(* Logix 5000 Rung export; software revision 16.03 *)

MODULES
   MNETCR : vendor None type None code None
   RemoteENBT_Slot6 : vendor None type None code None
END_MODULES

TYPE MNETCRCONTROL :   // Values used by program for data transfer operation between the module and the processor.
STRUCT
   BootTimer : TIMER;   // Timer used to clear both cold and warm boot requests
   WarmBoot : BOOL;   // Partial reset of the Module.
   ColdBoot : BOOL;   // Full reset of the Module.
   ResetStatus : BOOL;   // Resets module status
   EventCmdTrigger : BOOL;   // Initiates Event Command.
   EventCmdPending : BOOL;   // Allows Event Command.
   ClientID : INT;   // Client ID to poll a server with the Event Command.
   EventCmd : MNETCREVENTCMD;   // Holds Event Command configuration
   CmdControl : MNETCRCMDCONTROL;   // Holds Command Control status
   CmdControlTrigger : BOOL;   // Initiates Command Control.
   CmdControlPending : BOOL;   // Allows CmdControlTriger.
   IPAddress : MNETCRIPADDRESS;   // IP address statistics including triggers
   WriteCmdBits : INT[30];   // Selects individual clients to to activate its commands.
END_STRUCT
END_TYPE

TYPE MNETCRDATA :   // Contains Read Data (data read from the module to the processor) and Write Data (data written from the processor to the module)
STRUCT
   ReadData : INT[600];   // Data read from module
   WriteData : INT[600];   // Data to write to module
END_STRUCT
END_TYPE

TYPE MNETCREVENTCMD :   // Data structure to use for Event message generation.
STRUCT
   IP0 : INT;   // First digit of IP address
   IP1 : INT;   // Second digit of IP address
   IP2 : INT;   // Third digit of IP address
   IP3 : INT;   // Last digit of IP address
   ServPort : INT;   // TCP Service Port number (0-65535), 502 for MBAP, 2000 for MNET
   SlvAddrNode : INT;   // Modbus slave node address (0 to 247)
   DBAddress : INT;   // Module internal database to use with message
   Count : INT;   // Register or data point count
   Swap : INT;   // Swap code to use with functions 3 and 4
   MBFunction : INT;   // Modbus function code for message
   Address : INT;   // Address to interface with in device
END_STRUCT
END_TYPE

TYPE MNETCRIPADDRESS :   // This object holds IP address status with set IP & get IP triggers.
STRUCT
   IPgetTrigger : BOOL;   // Triggers get IP address.
   IPreceived : INT[4];   // Displays received IP address.
   IPsetTrigger : BOOL;   // Triggers set IP address
   IPrequested : INT[4];   // Displays requested IP address
END_STRUCT
END_TYPE

TYPE MNETCRMODULEDEF :   // This defines the whole module which includes all tags used in the program
STRUCT
   DATA : MNETCRDATA;   // Data read from module
   CONTROL : MNETCRCONTROL;   // MNETCR Module control
   STATUS : MNETCRSTATUS;   // Client ,Server Status and blocks status
   UTIL : MNETCRUTIL;   // Block statistics
END_STRUCT
END_TYPE

TYPE MNETCRUTIL :   // Values used by program for data transfer operation between the module and the processor.
STRUCT
   LastRead : INT;   // Index of last read block
   LastWrite : INT;   // Index of last write block
   BlockIndex : INT;   // Computed block offset for data table
   ReadDataSizeGet : INT;   // Gets ReadData Array Length.
   WriteDataSizeGet : INT;   // Gets WriteData Array Length.
   ReadDataBlkCount : INT;   // Holds the value of the Block Counts of the Read Data Array.
   WriteDataBlkCount : INT;   // Holds the value of the Block Counts of the Write Data Array.
   RBTSremainder : INT;   // Holds remainder calculation value from the read array.
   WBTSremainder : INT;   // Holds remainder calculation value from the write array.
   IPgetPending : BOOL;   // Allows setting IP
   IPsetPending : BOOL;   // Allowes getting IP
   InitOutBlkIDLim : INT;   // Block Index Limit for ReadData size of the array
END_STRUCT
END_TYPE

TYPE MNETCRBLOCKSTATS :   // This object is used to store the block transfer statistics for the MVI56-MNETCR module.
STRUCT
   Read : INT;   // Total number of read block transfers
   Write : INT;   // Total number of write block transfers
   Parse : INT;   // Total number of blocks parsed
   Event : INT;   // Total number of event blocks received
   Cmd : INT;   // Total number of command blocks received
   Err : INT;   // Total number of block transfer errors
END_STRUCT
END_TYPE

TYPE MNETCRCLIENTSTATS :   // This object is used to store the port statistics for an MVI56-MNETCR port.
STRUCT
   CmdReq : INT;   // Total number of command list requests sent
   CmdResp : INT;   // Total number of command list responses received
   CmdErr : INT;   // Total number of command list errors
   Requests : INT;   // Total number of requests for port
   Responses : INT;   // Total number of responses for port
   ErrSent : INT;   // Total number of errors sent
   ErrRec : INT;   // Total number of errors received
   CfgErrWord : INT;   // Configuration Error Word
   CurErr : INT;   // Current Error code
   LastErr : INT;   // Last recorded error code
END_STRUCT
END_TYPE

TYPE MNETCRCMDCONTROL :   // MVI56E-MNETCR Command Control
STRUCT
   ClientIDreq : INT;   // Requested Client ID.
   CmdQty : INT;   // Command Quantaty for the Client.
   CmdIndex : INT[16];   // Command Index per client. (0 to 15)
END_STRUCT
END_TYPE

TYPE MNETCRSTATUS :   // This status data is returned on each read block and can be used to detect proper module operation.
STRUCT
   PassCnt : INT;   // Program cycle counter
   BlockStats : MNETCRBLOCKSTATS;   // Block Statistics
   CmdBits : INT[30];   // Client Command Status.
   ClientStatsTrigger : BOOL;   // Get Client Status
   ClientIDReq : INT;   // Client ID requested.
   ClientStatus : MNETCRCLIENTSTATS[30];   // Client Status requests
   ClientIDRec : INT;   // Client ID received.
   CmdErrorList : INT[16];   // Cmd Error List
   ClientStatsPending : BOOL;   // Allows Get Client Status
END_STRUCT
END_TYPE

ADD_ON_INSTRUCTION AOI56MNETCR   (* revision 1.6, vendor ProSoft Technology Inc. *)
// Add-On for MVI56-MNETCR and  MVI56E-MNETCR Modules
// Revision note:
// v1.6 - Fixed copy length from 10 to 1 with client status logic
VAR_IN_OUT
   Connection_Input : INT[42]; {required}   // Input parameters.
   Connection_Output : INT[42]; {required}   // Output parameters.
   MNETCR : MNETCRMODULEDEF; {required}
END_VAR
VAR
   MJFAULTS : DINT[12];
END_VAR

ROUTINE Logic   (* ladder *)
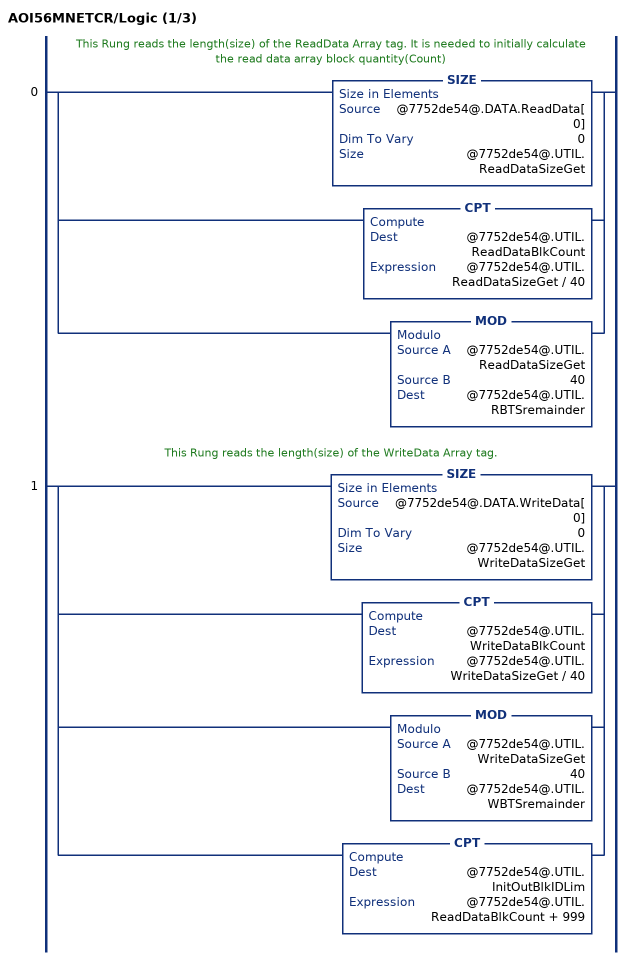
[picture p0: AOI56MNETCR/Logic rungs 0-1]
   // This Rung reads the length(size) of the ReadData Array tag. It is needed to initially calculate the read data array block quantity(Count)
   0: [SIZE(@7752de54@.DATA.ReadData[0],0,@7752de54@.UTIL.ReadDataSizeGet) ,CPT(@7752de54@.UTIL.ReadDataBlkCount,@7752de54@.UTIL.ReadDataSizeGet / 40) ,MOD(@7752de54@.UTIL.ReadDataSizeGet,40,@7752de54@.UTIL.RBTSremainder) ];
   // This Rung reads the length(size) of the WriteData Array tag.
   1: [SIZE(@7752de54@.DATA.WriteData[0],0,@7752de54@.UTIL.WriteDataSizeGet) ,CPT(@7752de54@.UTIL.WriteDataBlkCount,@7752de54@.UTIL.WriteDataSizeGet / 40) ,MOD(@7752de54@.UTIL.WriteDataSizeGet,40,@7752de54@.UTIL.WBTSremainder) ,CPT(@7752de54@.UTIL.InitOutBlkIDLim,@7752de54@.UTIL.ReadDataBlkCount + 999) ];
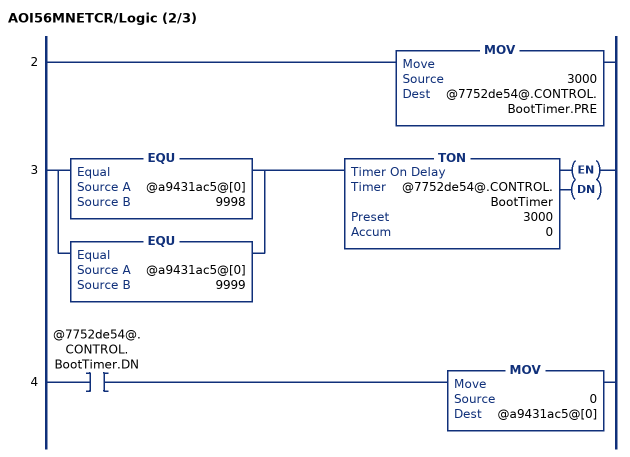
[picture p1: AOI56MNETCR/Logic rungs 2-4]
   2: MOV(3000,@7752de54@.CONTROL.BootTimer.PRE);
   3: [EQU(@a9431ac5@[0],9998) ,EQU(@a9431ac5@[0],9999) ]TON(@7752de54@.CONTROL.BootTimer,3000,0);
   4: XIC(@7752de54@.CONTROL.BootTimer.DN)MOV(0,@a9431ac5@[0]);
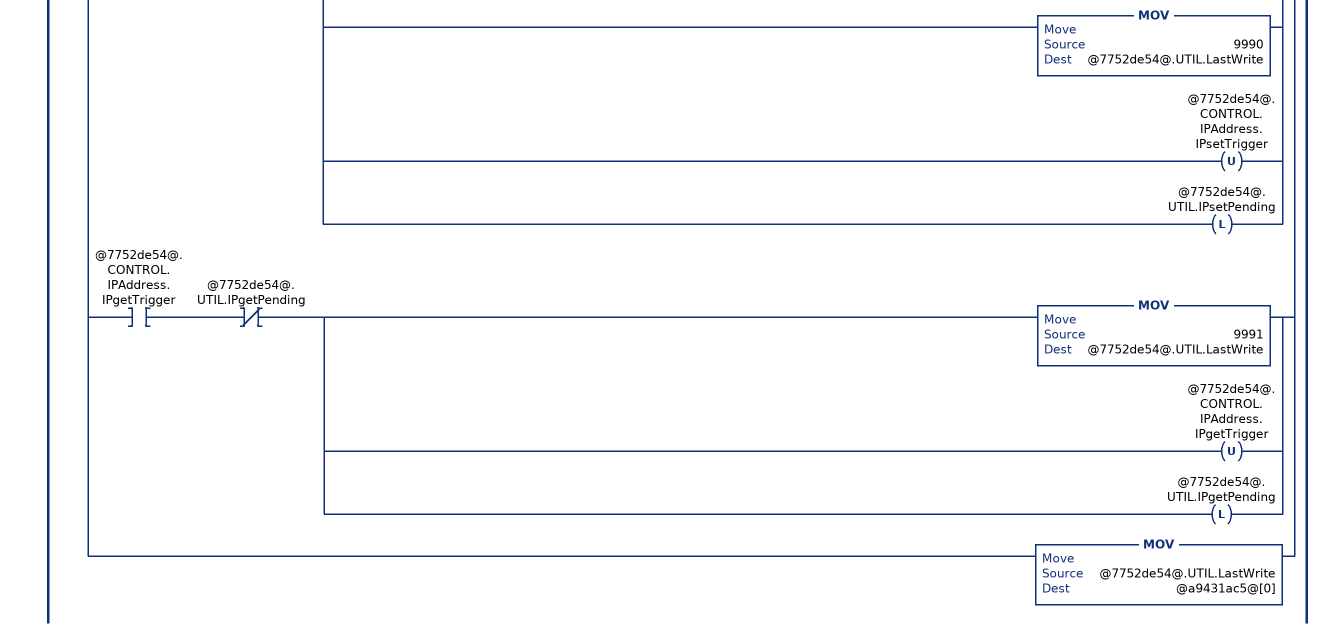
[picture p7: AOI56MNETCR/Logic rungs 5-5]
   // This rung is used to check for a new read block from the MVI56-MNETCR module in slot 1.  If new data is available, the LastRead and Data[41] will not be equal.  This will force the program to call the ReadData subroutine to process the new data received.  After the new data is placed in the Modbus Data Table, the program will send new data to the module using the WriteData subroutine.
   5: NEQ(@0dfc57aa@[41],@7752de54@.UTIL.LastRead)[MOV(@0dfc57aa@[41],@7752de54@.UTIL.LastRead) ,[EQU(-1,@7752de54@.UTIL.LastRead) ,EQU(0,@7752de54@.UTIL.LastRead) ] [MOV(@0dfc57aa@[1],@7752de54@.STATUS.PassCnt) ,COP(@0dfc57aa@[2],@7752de54@.STATUS.BlockStats.Read,6) ,COP(@0dfc57aa@[8],@7752de54@.STATUS.CmdBits[0],30) ] ,GEQ(@7752de54@.UTIL.LastRead,1) [LEQ(@7752de54@.UTIL.LastRead,@7752de54@.UTIL.ReadDataBlkCount) [CPT(@7752de54@.UTIL.BlockIndex,(@7752de54@.UTIL.LastRead - 1) * 40) ,COP(@0dfc57aa@[1],@7752de54@.DATA.ReadData[@7752de54@.UTIL.BlockIndex],40) ] ,CMP(@7752de54@.UTIL.LastRead - @7752de54@.UTIL.ReadDataBlkCount = 1) GRT(@7752de54@.UTIL.RBTSremainder,0) [CPT(@7752de54@.UTIL.BlockIndex,(@7752de54@.UTIL.LastRead - 1) * 40) ,COP(@0dfc57aa@[1],@7752de54@.DATA.ReadData[@7752de54@.UTIL.BlockIndex],@7752de54@.UTIL.RBTSremainder) ] ] ,LIM(2000,@7752de54@.UTIL.LastRead,2029) EQU(@0dfc57aa@[1],1) OTU(@7752de54@.CONTROL.EventCmdPending) ,LIM(3000,@7752de54@.UTIL.LastRead,3029) [MOV(@0dfc57aa@[1],@7752de54@.STATUS.ClientIDRec) ,SUB(@7752de54@.STATUS.ClientIDRec,3000,@7752de54@.STATUS.ClientIDRec) ,COP(@0dfc57aa@[2],@7752de54@.STATUS.ClientStatus[@7752de54@.STATUS.ClientIDRec],1) ,COP(@0dfc57aa@[12],@7752de54@.STATUS.CmdErrorList[0],16) ,OTU(@7752de54@.STATUS.ClientStatsPending) ] ,LIM(5001,@7752de54@.UTIL.LastRead,5016) LIM(1,@0dfc57aa@[1],16) OTU(@7752de54@.CONTROL.CmdControlPending) ,EQU(@7752de54@.UTIL.LastRead,9990) [COP(@0dfc57aa@[1],@7752de54@.CONTROL.IPAddress.IPrequested[0],4) ,OTU(@7752de54@.UTIL.IPsetPending) ] ,EQU(@7752de54@.UTIL.LastRead,9991) [COP(@0dfc57aa@[1],@7752de54@.CONTROL.IPAddress.IPreceived[0],4) ,OTU(@7752de54@.UTIL.IPgetPending) ] ,MOV(@0dfc57aa@[0],@7752de54@.UTIL.LastWrite) ,XIC(@7752de54@.CONTROL.ResetStatus) [MOV(9997,@7752de54@.UTIL.LastWrite) ,OTU(@7752de54@.CONTROL.ResetStatus) ] ,XIC(@7752de54@.CONTROL.WarmBoot) [MOV(9998,@7752de54@.UTIL.LastWrite) ,OTU(@7752de54@.CONTROL.WarmBoot) ] ,XIC(@7752de54@.CONTROL.ColdBoot) [MOV(9999,@7752de54@.UTIL.LastWrite) ,OTU(@7752de54@.CONTROL.ColdBoot) ] ,GEQ(@7752de54@.UTIL.LastWrite,1) [LEQ(@7752de54@.UTIL.LastWrite,@7752de54@.UTIL.WriteDataBlkCount) [CPT(@7752de54@.UTIL.BlockIndex,(@7752de54@.UTIL.LastWrite - 1) * 40) ,COP(@7752de54@.DATA.WriteData[@7752de54@.UTIL.BlockIndex],@a9431ac5@[1],40) ] ,CMP(@7752de54@.UTIL.LastWrite - @7752de54@.UTIL.WriteDataBlkCount = 1) GRT(@7752de54@.UTIL.WBTSremainder,0) [CPT(@7752de54@.UTIL.BlockIndex,(@7752de54@.UTIL.LastWrite - 1) * 40) ,COP(@7752de54@.DATA.WriteData[@7752de54@.UTIL.BlockIndex],@a9431ac5@[1],@7752de54@.UTIL.WBTSremainder) ] ] ,[EQU(-1,@7752de54@.UTIL.LastWrite) ,EQU(0,@7752de54@.UTIL.LastWrite) ] COP(@7752de54@.CONTROL.WriteCmdBits[0],@a9431ac5@[1],30) ,LIM(1000,@7752de54@.UTIL.LastWrite,1124) [LEQ(@7752de54@.UTIL.LastWrite,@7752de54@.UTIL.InitOutBlkIDLim) [CPT(@7752de54@.UTIL.BlockIndex,(@7752de54@.UTIL.LastWrite - 1000) * 40) ,COP(@7752de54@.DATA.ReadData[@7752de54@.UTIL.BlockIndex],@a9431ac5@[1],40) ] ,GRT(@7752de54@.UTIL.LastWrite,@7752de54@.UTIL.InitOutBlkIDLim) FLL(0,@a9431ac5@[1],40) ] ,XIC(@7752de54@.CONTROL.EventCmdTrigger) XIO(@7752de54@.CONTROL.EventCmdPending) [COP(@7752de54@.CONTROL.EventCmd.IP0,@a9431ac5@[1],11) ,LIM(0,@7752de54@.CONTROL.ClientID,29) ADD(2000,@7752de54@.CONTROL.ClientID,@7752de54@.UTIL.LastWrite) ,OTU(@7752de54@.CONTROL.EventCmdTrigger) ,OTL(@7752de54@.CONTROL.EventCmdPending) ] ,XIC(@7752de54@.STATUS.ClientStatsTrigger) XIO(@7752de54@.STATUS.ClientStatsPending) [LIM(0,@7752de54@.STATUS.ClientIDreq,29) ADD(3000,@7752de54@.STATUS.ClientIDreq,@7752de54@.UTIL.LastWrite) ,OTU(@7752de54@.STATUS.ClientStatsTrigger) ,OTL(@7752de54@.STATUS.ClientStatsPending) ] ,XIC(@7752de54@.CONTROL.CmdControlTrigger) XIO(@7752de54@.CONTROL.CmdControlPending) [LIM(0,@7752de54@.CONTROL.CmdControl.ClientIDreq,29) MOV(@7752de54@.CONTROL.CmdControl.ClientIDreq,@a9431ac5@[1]) ,COP(@7752de54@.CONTROL.CmdControl.CmdIndex[0],@a9431ac5@[2],16) ,LIM(1,@7752de54@.CONTROL.CmdControl.CmdQty,16) ADD(5000,@7752de54@.CONTROL.CmdControl.CmdQty,@7752de54@.UTIL.LastWrite) ,OTU(@7752de54@.CONTROL.CmdControlTrigger) ,OTL(@7752de54@.CONTROL.CmdControlPending) ] ,XIC(@7752de54@.CONTROL.IPAddress.IPsetTrigger) XIO(@7752de54@.UTIL.IPsetPending) [COP(@7752de54@.CONTROL.IPAddress.IPrequested[0],@a9431ac5@[1],4) ,MOV(9990,@7752de54@.UTIL.LastWrite) ,OTU(@7752de54@.CONTROL.IPAddress.IPsetTrigger) ,OTL(@7752de54@.UTIL.IPsetPending) ] ,XIC(@7752de54@.CONTROL.IPAddress.IPgetTrigger) XIO(@7752de54@.UTIL.IPgetPending) [MOV(9991,@7752de54@.UTIL.LastWrite) ,OTU(@7752de54@.CONTROL.IPAddress.IPgetTrigger) ,OTL(@7752de54@.UTIL.IPgetPending) ] ,MOV(@7752de54@.UTIL.LastWrite,@a9431ac5@[0]) ];
END_ROUTINE

ROUTINE Prescan   (* ladder *)
// Prescan
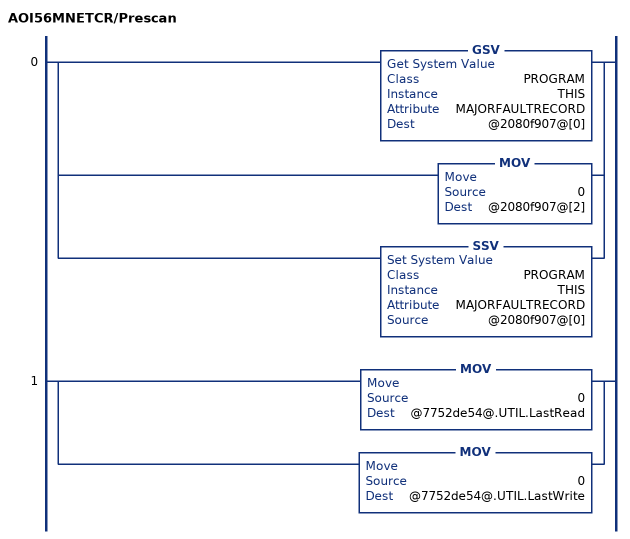
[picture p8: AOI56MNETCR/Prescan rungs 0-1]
   0: [GSV(PROGRAM,THIS,MAJORFAULTRECORD,@2080f907@[0]) ,MOV(0,@2080f907@[2]) ,SSV(PROGRAM,THIS,MAJORFAULTRECORD,@2080f907@[0]) ];
   1: [MOV(0,@7752de54@.UTIL.LastRead) ,MOV(0,@7752de54@.UTIL.LastWrite) ];
END_ROUTINE
END_ADD_ON_INSTRUCTION

VAR_GLOBAL   (* controller tags *)
   RemoteENBT_Slot6:1:O : AB:1756_MODULE_INT_84Bytes:O:0;
   MNETCR : MNETCRMODULEDEF;
        .BLK2000CLIENTID   // Client's Index ID.
        .BLK3000CLIENTID   // Holds Block 3000 Client ID
        .BLK5000CLIENTID   // Holds Block 5000 Client ID
        .BLK_1CLIENTID   // Holds Client ID for Command Bits Control.
        .BP.LASTREAD   // Index of last read block
        .BP.LASTWRITE   // Holds the value to be written on the last scan.
        .CMDCNTRL   // Initiates Command Control
        .COLDBOOT   // Re-initializes all the module's parameters
        .EVENTCMD   // Initiates an Event.
        .GETCLNTSTAT   // Initiates retreaval of Client Status.
        .GETIPADDRESS   // Initiates the retreaval of IP Address from the module.
        .HALTCLNTSTAT   // Halts Client Status Retreaval until the Module is ready for the next Status Retreaval.
        .HALTCMDBITCNTRL   // Halts Command Control Bits execution until the Module is ready for the next Command.
        .HALTCMDCNTRL   // Halts Command Control until the Module is ready for the next Command.
        .HALTEVENTCMD   // Halts Event Initiation until the Module is ready for the next Event.
        .HALTGETIPADDR   // Halts the IP Retreaval until the module is ready.
        .HALTSETIPADDRESS   // Halts the IP Adress Setting until the Module is ready for it.
        .INSTAT.CMDERRORLIST[0]   // Reads Command related errors
        .READIPADDRESS.IP[0]   // Reads Module's set IP Address
        .SETIPADDRESS   // Initiates the setting of the IP Address for the module.
        .WARMBOOT   // Re-loads MNET.CFG file
        .WRITEIPADDRESSACK.IP[0]   // Ack. from the module that it has received the new IP Address
   AOI56MNETCR : AOI56MNETCR;
   RemoteENBT_Slot6:1:I : AB:1756_MODULE_INT_84Bytes:I:0;
END_VAR

PROGRAM MainProgram

ROUTINE MainRoutine   (* ladder *)
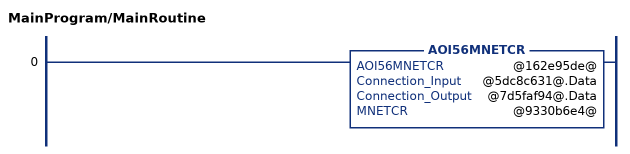
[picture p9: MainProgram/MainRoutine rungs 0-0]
   0: AOI56MNETCR(@162e95de@,@5dc8c631@.Data,@7d5faf94@.Data,@9330b6e4@);
END_ROUTINE
END_PROGRAM
